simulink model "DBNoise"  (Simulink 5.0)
settings: Solver=FixedStepDiscrete  SolverMode=SingleTasking  StartTime=t0  StopTime=tfin  RelTol=1e-3  AbsTol=1e-6
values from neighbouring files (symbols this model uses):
  Ou = 3    [demo_DBNoise.m]
  Sw = 0.01    [demo_DBNoise.m]

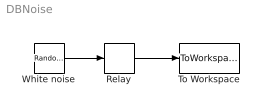
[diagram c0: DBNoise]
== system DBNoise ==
  Relay : Relay  OnSwitchValue=Sw  OffSwitchValue=-Sw  OnOutputValue=-Ou  OffOutputValue=Ou  ShowAdditionalParam=on
  To Workspace : ToWorkspace  VariableName=u  SampleTime=-1  SaveFormat=Array
  White noise : RandomNumber  Seed=1024  SampleTime=0
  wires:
  White noise/1 -> Relay/1
  Relay/1 -> To Workspace/1
